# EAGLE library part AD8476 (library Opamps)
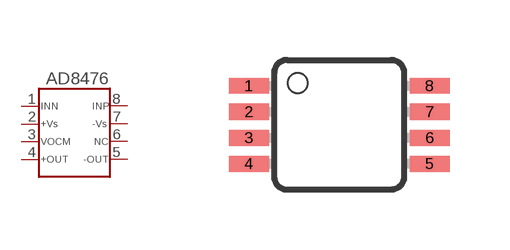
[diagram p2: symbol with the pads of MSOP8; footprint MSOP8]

Designator prefix U

## AD8476  [MSOP8]
1  1  in
2  2  in
3  3  in
4  4  out
5  5  out
6  6  nc
7  7  in
8  8  in

## Footprint MSOP8 (pad centres in mm)
smd 1 x 0.4: 1 -2.263,0.976; 2 -2.263,0.326; 3 -2.263,-0.324; 4 -2.263,-0.974; 5 2.262,-0.974; 6 2.262,-0.324; 7 2.262,0.326; 8 2.262,0.976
